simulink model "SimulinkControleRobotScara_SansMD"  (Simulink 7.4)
settings: Solver=ode45  StartTime=0.0  StopTime=T  FixedStep=0.1  MaxStep=0.1  MinStep=0.01  RelTol=0.1  AbsTol=0.01
libraries: simulink x3

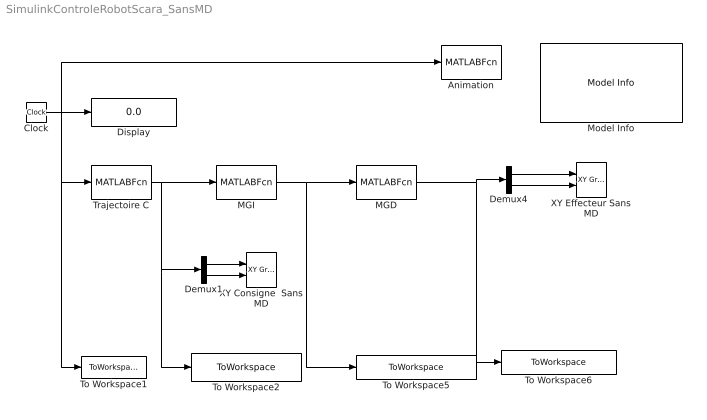
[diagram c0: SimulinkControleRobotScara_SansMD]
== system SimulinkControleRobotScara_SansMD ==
  Animation : MATLABFcn  Tag=Affichage  Description=Affichage  MATLABFcn=SetAffichage  OutputDimensions=0
  Clock : Clock
  Demux1 : Demux  Outputs=2
  Demux4 : Demux  Outputs=2
  Display : Display
  MGD : MATLABFcn  MATLABFcn=ModeleGeometriqueDirect  OutputDimensions=2
  MGI : MATLABFcn  MATLABFcn=ModeleGeometriqueInverse  OutputDimensions=2
  Model Info : simulink/Model-Wide Utilities/Model Info  SystemSampleTime=-1  InitialBlockCM=None  BlockCM=None  Frame=on  DisplayStringWithTags=|  HorizontalTextAlignment=Left  LeftAlignmentValue=0.02  SourceBlockDiagram=SimulinkControleRobotScara_SansMD  TagMaxNumber=20
      | Asservissement de position 
      | d'un robot SCARA 2D RR
      | 
      | Lounis Adouane
      | Polytech'Clermont-Ferrand
  To Workspace1 : ToWorkspace  VariableName=DS_Temps  SaveFormat=Array
  To Workspace2 : ToWorkspace  VariableName=DS_PositionConsigne  SaveFormat=Array
  To Workspace5 : ToWorkspace  VariableName=DS_ThetaArticulations  SaveFormat=Array
  To Workspace6 : ToWorkspace  VariableName=DS_PositionEffecteur  SaveFormat=Array
  Trajectoire C : MATLABFcn  MATLABFcn=TrajectoireConsigne  OutputDimensions=2
  XY Consigne  Sans MD : simulink/Sinks/XY Graph  SystemSampleTime=-1  xmin=-15  xmax=15  ymin=-15  ymax=15  st=-1
  XY Effecteur Sans MD : simulink/Sinks/XY Graph  SystemSampleTime=-1  xmin=-15  xmax=15  ymin=-15  ymax=15  st=-1
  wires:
  Clock/1 -> Display/1, To Workspace1/1, Animation/1, Trajectoire C/1
  Trajectoire C/1 -> Demux1/1, To Workspace2/1, MGI/1
  Demux1/1 -> XY Consigne  Sans MD/1
  Demux1/2 -> XY Consigne  Sans MD/2
  Demux4/1 -> XY Effecteur Sans MD/1
  Demux4/2 -> XY Effecteur Sans MD/2
  MGD/1 -> To Workspace6/1, Demux4/1
  MGI/1 -> To Workspace5/1, MGD/1
